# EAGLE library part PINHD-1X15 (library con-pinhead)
PIN HEADER
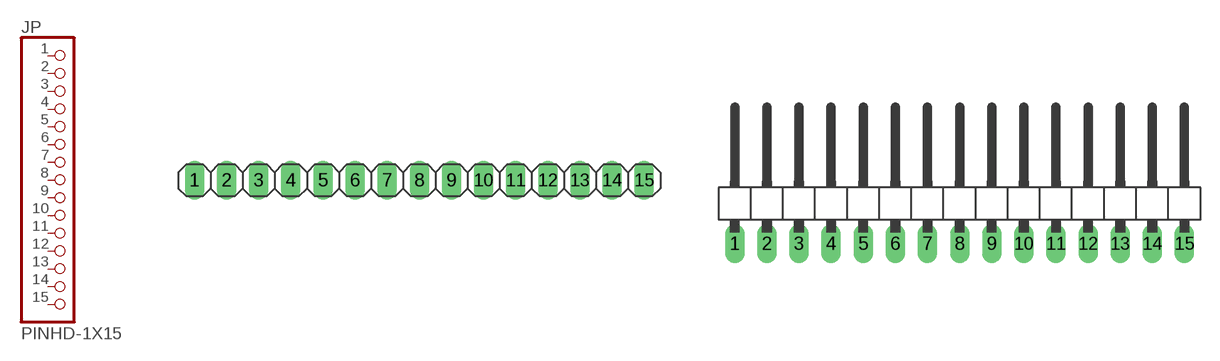
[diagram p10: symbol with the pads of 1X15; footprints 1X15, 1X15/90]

Designator prefix JP

## PINHD-1X15_2.54  [1X15]
1  1  pas
2  2  pas
3  3  pas
4  4  pas
5  5  pas
6  6  pas
7  7  pas
8  8  pas
9  9  pas
10  10  pas
11  11  pas
12  12  pas
13  13  pas
14  14  pas
15  15  pas

## PINHD-1X15_2.54-90°  [1X15/90]
Pads as for 1X15

## PINHD-1X15_2.00  [1X15M]
Pads as for 1X15

## PINHD-1X15_2.54-SMD  [1X15SMD]
Pads as for 1X15

## PINHD-1X15_2.54-SMD-90°  [1X15SMD/90]
Pads as for 1X15

## Footprint 1X15 (pad centres in mm)
PIN HEADER - 2.54
drill 1.016 long: 1 -17.78,0; 2 -15.24,0; 3 -12.7,0; 4 -10.16,0; 5 -7.62,0; 6 -5.08,0; 7 -2.54,0; 8 0,0; 9 2.54,0; 10 5.08,0; 11 7.62,0; 12 10.16,0; 13 12.7,0; 14 15.24,0; 15 17.78,0

## Footprint 1X15/90 (pad centres in mm)
PIN HEADER - 2.54 90°
drill 1.016 long: 1 -17.78,-3.81; 2 -15.24,-3.81; 3 -12.7,-3.81; 4 -10.16,-3.81; 5 -7.62,-3.81; 6 -5.08,-3.81; 7 -2.54,-3.81; 8 0,-3.81; 9 2.54,-3.81; 10 5.08,-3.81; 11 7.62,-3.81; 12 10.16,-3.81; 13 12.7,-3.81; 14 15.24,-3.81; 15 17.78,-3.81

## Footprint 1X15M (pad centres in mm)
PIN HEADER - 2
drill 0.914 square: 1 -14,0
drill 0.914: 2 -12,0; 3 -10,0; 4 -8,0; 5 -6,0; 6 -4,0; 7 -2,0; 8 0,0; 9 2,0; 10 4,0; 11 6,0; 12 8,0; 13 10,0; 14 12,0; 15 14,0

## Footprint 1X15SMD (pad centres in mm)
PIN HEADER - 2.54 SMD
smd 1.016 x 3.302: 1 -1.27,1.27; 2 1.27,-1.27; 3 3.81,1.27; 4 6.35,-1.27; 5 8.89,1.27; 6 11.43,-1.27; 7 13.97,1.27; 8 16.51,-1.27; 9 19.05,1.27; 10 21.59,-1.27; 11 24.13,1.27; 12 26.67,-1.27; 13 29.21,1.27; 14 31.75,-1.27; 15 34.29,1.27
